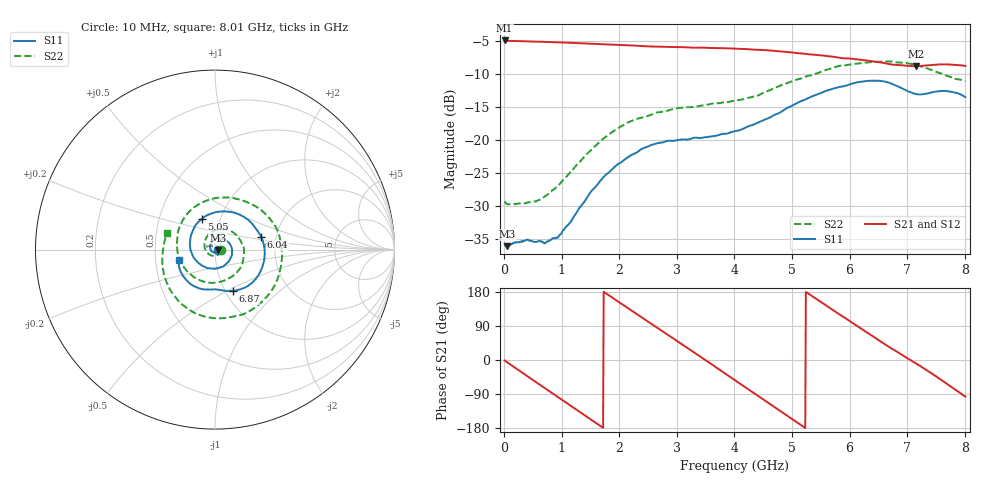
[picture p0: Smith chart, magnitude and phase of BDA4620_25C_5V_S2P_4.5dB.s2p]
!Agilent Technologies,E5071B,MY42404982,A.09.10
!Date: Wed May 06 08:59:02 2026
!Data & Calibration Information:
!Freq	S11:SOLT2(ON)	S21:SOLT2(ON)	S12:SOLT2(ON)	S22:SOLT2(ON)
# Hz S RI R 50
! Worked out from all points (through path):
!   801 points, 10 MHz to 8.01 GHz, reference 50 ohm
!   highest |S21| = -4.95 dB at 10 MHz (marker M1); lowest = -8.8 dB at 7.15 GHz (marker M2)
!   group delay of S21, straight-line fit = 283 ps
!   lowest |S11| = -36.0 dB at 60 MHz (marker M3), VSWR 1.03, Z = 51.6 - j0.136 ohm
!   |S11| at or under -10 dB: start of sweep to end of sweep
!   |S22| runs from -29.7 to -8.1 dB; largest |S21 - S12| = 0.0023
!   S11 on the Smith chart (normalised r, x): 10 MHz: 1.03, -0.00; 5.05 GHz: 0.82, +0.29; 6.04 GHz: 1.67, +0.26; 6.87 GHz: 1.08, -0.53; 8.01 GHz: 0.66, -0.08
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1e7  0.0164 -0.000983  0.5657 -0.0121  0.5662 -0.0124  0.0343 -0.0027
6e7  0.0157 -0.00131  0.5596 -0.0643  0.5606 -0.0656  0.0323 -0.00578
3.7e8  0.0142 -0.01  0.4328 -0.3512  0.4331 -0.3521  0.019 -0.0275
7.3e8  -0.000102 -0.0169  0.1274 -0.5366  0.1272 -0.537  -0.0173 -0.0339
1.03e9  -0.0188 -0.00896  -0.1667 -0.5192  -0.1672 -0.5196  -0.0494 -0.00919
1.35e9  -0.0278 0.0166  -0.4185 -0.339  -0.4189 -0.3398  -0.0572 0.0424
1.65e9  -0.0147 0.0456  -0.5258 -0.0752  -0.5267 -0.0754  -0.0265 0.0922
1.94e9  0.017 0.0615  -0.4878 0.1932  -0.4885 0.1935  0.0351 0.1148
2.32e9  0.0664 0.0474  -0.2531 0.4496  -0.2539 0.4499  0.1226 0.0779
2.68e9  0.0951 -0.00102  0.0618 0.5044  0.0624 0.5048  0.1618 -0.0097
2.99e9  0.0844 -0.0529  0.3138 0.3954  0.3147 0.3949  0.1434 -0.0978
3.39e9  0.0325 -0.0984  0.4906 0.0931  0.4912 0.0921  0.0417 -0.1757
4.01e9  -0.0836 -0.0814  0.2934 -0.3932  0.2934 -0.394  -0.1683 -0.1051
4.5e9  -0.1396 0.0215  -0.1166 -0.4648  -0.1174 -0.4652  -0.2069 0.0946
5.05e9  -0.074 0.1708  -0.4316 -0.1485  -0.4323 -0.1476  -0.0188 0.2822
5.35e9  0.0276 0.2125  -0.4336 0.0885  -0.4336 0.0891  0.1407 0.277
6.04e9  0.2571 0.0716  -0.063 0.4066  -0.0625 0.4073  0.3735 -0.0193
6.68e9  0.1767 -0.2067  0.3081 0.2144  0.3093 0.2143  0.1827 -0.3482
6.87e9  0.0989 -0.2303  0.3519 0.1096  0.3528 0.1086  0.0654 -0.3799
7.15e9  0.0141 -0.2223  0.3569 -0.0562  0.3576 -0.057  -0.1155 -0.352
7.57e9  -0.1092 -0.2073  0.2375 -0.2879  0.2379 -0.289  -0.2784 -0.1585
8.01e9  -0.2022 -0.0604  -0.0429 -0.3605  -0.0436 -0.3618  -0.2662 0.0902
